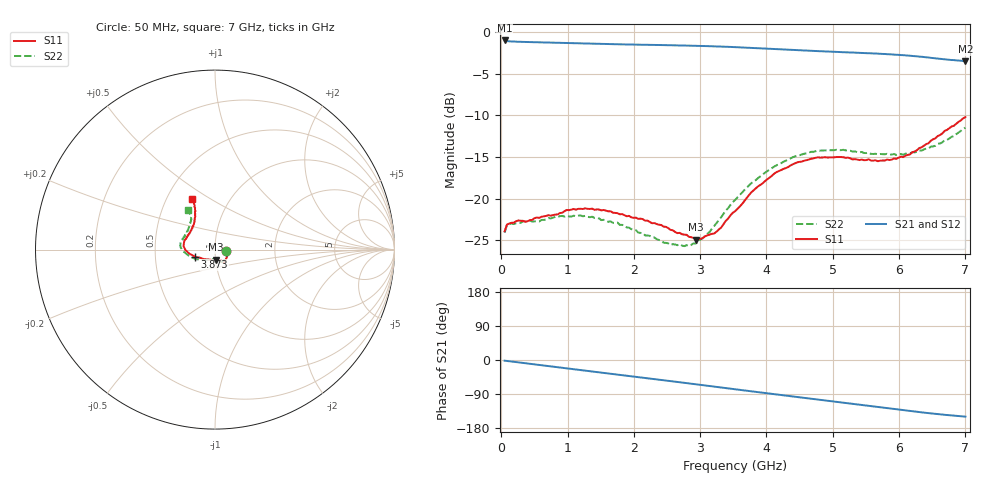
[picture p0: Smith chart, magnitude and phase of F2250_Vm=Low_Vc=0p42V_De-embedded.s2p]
! Integrated Device Technology
! Corporate Headquarters
! 6024 Silver Creek Valley Road
! San Jose, CA 95138  USA
! Phone:  1-408-284-8200
! Toll Free:  1-800-223-1366
! Webpage:  http://www.idt.com/
! Timing and RF Division
! 515 Groton Road, Suite 102
! Westford, MA 01886-6024
! Device:  F2250
! Description: Voltage Variable RF Attenuator
! Frequency:  50.0 -  6000.00 MHz
! Package:  3x3 mm Thin QFN Plastic Package: 16 pin
! Ports:  2 RF, 3 DC
!  Pin  1  = GND
!  Pin  2  = NC
!  Pin  3  = RF1  = Port 1
!  Pin  4  = NC
!  Pin  5  = GND
!  Pin  6  = GND
!  Pin  7  = GND
!  Pin  8  = GND
!  Pin  9  = NC
!  Pin 10  = RF2  = Port 2
!  Pin 11  = NC
!  Pin 12  = GND
!  Pin 13  = GND
!  Pin 14  = VCNTRL
!  Pin 15  = VDD
!  Pin 16  = VMODE
! Vcntrl:  0.420 Volts
! Vmode:  +0.000 Volts
! Vdd:  +3.30  Volts
! Current:  1.125 mA
! Data:  The device was measured on a the F2250 evaluation board which has
!  individual transmission lines to the RF pins.  Data was collected
!  using a calibrated network analyzer.  The evaluation board was
!  de-embedded using a TRL calibration technique.
!  The reference plane is the edge of the package pin.
! Misc:  SN 10
!  Action Tracker AT0258
! Date Measured:  2014-11-26
! Date:  2015-10-15  MJV
! Note:
!  Integrated Device Technology supplies this data as a sample of measured
!  data at the package pin for this product.  Your particular data for this
!  product may vary.
!  Data was taken at 25 degrees C.
!  Integrated Device Technology reserves the right to change this data at anytime.
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# GHz S dB R 50
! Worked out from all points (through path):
!   201 points, 50 MHz to 7 GHz, reference 50 ohm
!   highest |S21| = -1.01 dB at 50 MHz (marker M1); lowest = -3.5 dB at 7 GHz (marker M2)
!   group delay of S21, straight-line fit = 60 ps
!   lowest |S11| = -24.9 dB at 2.934 GHz (marker M3), VSWR 1.12, Z = 50.1 - j5.69 ohm
!   |S11| at or under -10 dB: start of sweep to end of sweep
!   |S22| runs from -25.7 to -11.5 dB; largest |S21 - S12| = 0.00041
!   S11 on the Smith chart (normalised r, x): 50 MHz: 1.13, -0.02; 3.873 GHz: 0.80, -0.06; 7 GHz: 0.67, +0.42
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0.05  -23.93 -8.7  -1.01 -1.8  -1.00 -1.8  -24.09 -9.3
0.08475  -23.13 -8.5  -1.08 -2.5  -1.08 -2.5  -23.23 -8.6
0.15425  -22.91 -10.7  -1.13 -4.0  -1.13 -4.0  -23.00 -10.3
0.57125  -22.32 -27.6  -1.23 -13.1  -1.23 -13.1  -22.76 -29.1
0.71025  -21.99 -35.3  -1.26 -16.2  -1.26 -16.2  -22.35 -36.9
1.2315  -21.25 -52.4  -1.37 -27.4  -1.37 -27.4  -22.12 -57.6
1.75275  -21.75 -59.1  -1.46 -38.5  -1.46 -38.5  -22.88 -65.5
2.37825  -23.14 -60.3  -1.55 -51.8  -1.55 -51.8  -24.97 -69.4
2.552  -23.76 -64.2  -1.58 -55.6  -1.58 -55.7  -25.58 -75.2
2.83  -24.59 -77.8  -1.63 -61.7  -1.63 -61.7  -25.70 -93.1
2.93425  -24.92 -85.8  -1.65 -64.0  -1.65 -64.0  -25.40 -101.2
3.21225  -24.18 -114.3  -1.71 -70.2  -1.71 -70.2  -23.27 -125.8
3.525  -21.52 -142.5  -1.81 -77.1  -1.81 -77.1  -20.18 -144.7
3.8725  -18.53 -160.3  -1.94 -84.8  -1.94 -84.8  -17.54 -160.3
4.1505  -16.82 -170.6  -2.05 -90.9  -2.05 -90.9  -16.00 -170.4
4.39375  -15.89 -177.6  -2.14 -96.1  -2.14 -96.1  -15.04 -177.0
4.7065  -15.17 174.6  -2.26 -102.9  -2.26 -102.9  -14.38 176.3
5.15825  -15.04 163.8  -2.42 -112.7  -2.42 -112.7  -14.14 167.0
5.85325  -15.36 140.5  -2.67 -127.6  -2.67 -127.6  -14.74 151.7
6.166  -14.68 129.2  -2.84 -134.4  -2.84 -134.4  -14.57 142.8
6.444  -13.36 120.6  -3.05 -140.2  -3.05 -140.2  -13.98 133.4
7  -10.21 114.0  -3.49 -149.5  -3.49 -149.5  -11.48 123.9
